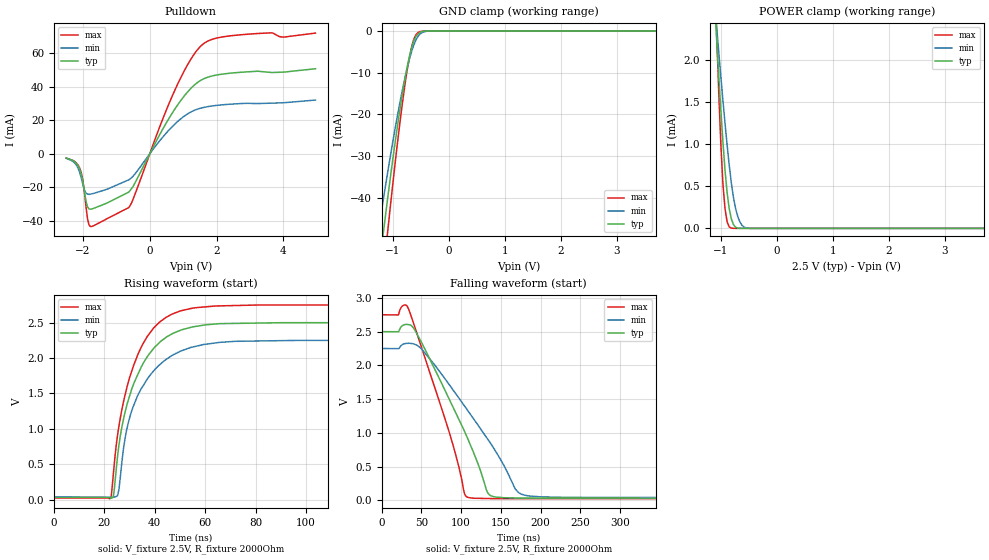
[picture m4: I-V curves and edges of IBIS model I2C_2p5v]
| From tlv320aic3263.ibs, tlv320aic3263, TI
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|   I2C_2p5v
[Model]   I2C_2p5v
Model_type   I/O_open_drain
Polarity   Non-Inverting
Enable   Active-High
Vinl = 0.75
Vinh = 1.75
Vmeas = 1.25
Vref = 0
Cref = 5pF
Rref = 2000
|   typ   min   max
C_comp   1.274pF   1.219pF   1.333pF
[Voltage Range]   2.5   2.25   2.75
[Temperature Range]   27   125   -40
[Pullup Reference]   2.5   2.25   2.75
[Pulldown Reference]   -0   -0   -0
[Power Clamp Reference]   2.5   2.25   2.75
[GND Clamp Reference]   -0   -0   -0
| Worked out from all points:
|   slope of the pulldown table from 0 to 0.375 V, typ, clamps not added: 26.4 ohm
|   GND clamp passes 1 mA (typ) near -0.57 V on its own axis
|   POWER clamp passes 1 mA (typ) near -0.96 V on its own axis
|   falling waveform, V_fixture 2.5V, R_fixture 2000Ohm: 20-80 % time 57.5ns typ, 76.1ns min, 43.6ns max; typ from 2.5 V to 0.031 V
|   rising waveform, V_fixture 2.5V, R_fixture 2000Ohm: 20-80 % time 11.8ns typ, 12.5ns min, 11.3ns max; typ from 0.031 V to 2.5 V
[Pulldown]
|   Voltage   I(typ)   I(min)   I(max)
-2.5V     -2.526mA   -2.66mA    -2.537mA
-2.237V   -4.926mA   -5.666mA   -4.77mA
-2.087V   -9.625mA   -11.74mA   -9.035mA
-2.013V   -15.52mA   -17.53mA   -14.79mA
-1.9V     -28.98mA   -23.51mA   -33.15mA
-1.825V   -32.66mA   -24.09mA   -41.94mA
-1.675V   -32.39mA   -23.49mA   -42.71mA
-625mV    -22.72mA   -15.42mA   -31.93mA
725mV     25.83mA    17.19mA    36.69mA
1.55V     43.97mA    27.3mA     64.52mA
2.525V    48.19mA    29.68mA    70.44mA
4.963V    50.63mA    32mA       71.83mA
[GND Clamp]
|   Voltage   I(typ)   I(min)   I(max)
-2.5V     -395.5mA   -330.9mA   -444.7mA
-1.375V   -71.35mA   -58.36mA   -85.71mA
-1.188V   -50.16mA   -41.75mA   -60.29mA
-1.15V    -46.08mA   -38.56mA   -55.36mA
-1.113V   -42.07mA   -35.43mA   -50.5mA
-1.075V   -38.14mA   -32.35mA   -45.71mA
-887.5mV  -19.93mA   -18.02mA   -23.34mA
-737.5mV  -8.099mA   -8.458mA   -8.701mA
-625mV    -2.309mA   -3.27mA    -1.918mA
-550mV    -742.7uA   -1.242mA   -338.4uA
-287.5mV  -254.6nA   -5.008uA   -31.57nA
4.963V    0A         0A         0A
[POWER Clamp]
|   Voltage   I(typ)   I(min)   I(max)
-2.5V     20.66mA    14.8mA     34.71mA
-1.113V   2.682mA    2.698mA    3.063mA
-1.075V   2.242mA    2.395mA    2.317mA
-1V       1.406mA    1.805mA    1mA
-962.5mV  1.026mA    1.521mA    525.7uA
-925mV    689.7uA    1.247mA    231.4uA
-887.5mV  420.9uA    988.2uA    76.84uA
-812.5mV  113.7uA    540.4uA    3.319uA
-700mV    3.918uA    146.5uA    40.28nA
-625mV    247.3nA    39.26uA    0A
-512.5mV  0A         2.416uA    0A
4.963V    0A         0A         0A
[Ramp]
R_load = 2000
|   typ   min   max
dV/dt_r   1.48138/1.18177e-008   1.32568/1.24678e-008   1.63535/1.12722e-008
dV/dt_f   1.48139/5.7451e-008   1.32569/7.60824e-008   1.63535/4.35846e-008
[Falling Waveform]
V_fixture = 2.5V
V_fixture_min = 2.25V
V_fixture_max = 2.75V
R_fixture = 2000Ohm
C_fixture = 0F
|   Time   V(typ)   V(min)   V(max)
0s        2.5V       2.25V      2.75V
33.44ns   2.604V     2.327V     2.844V
50.29ns   2.335V     2.241V     2.258V
85.86ns   1.476V     1.7V       973.4mV
104.3ns   1.019V     1.396V     94.24mV
107.1ns   945.1mV    1.35V      51.42mV
133.6ns   106.2mV    901.3mV    26.95mV
168ns     35.18mV    167.6mV    25.37mV
176.8ns   33.5mV     86.17mV    25.34mV
470ns     31.02mV    40.52mV    24.42mV
[Rising Waveform]
V_fixture = 2.5V
V_fixture_min = 2.25V
V_fixture_max = 2.75V
R_fixture = 2000Ohm
C_fixture = 0F
|   Time   V(typ)   V(min)   V(max)
0s        31.02mV    40.52mV    24.42mV
22.61ns   24.73mV    36.32mV    22.9mV
23.85ns   103.7mV    36.09mV    457.1mV
25.36ns   639.4mV    67.87mV    931.3mV
26.72ns   976.1mV    445.2mV    1.224V
29.13ns   1.358V     1.027V     1.608V
33.44ns   1.779V     1.484V     2.061V
41.98ns   2.223V     1.906V     2.509V
54.82ns   2.439V     2.154V     2.703V
470ns     2.5V       2.25V      2.75V
